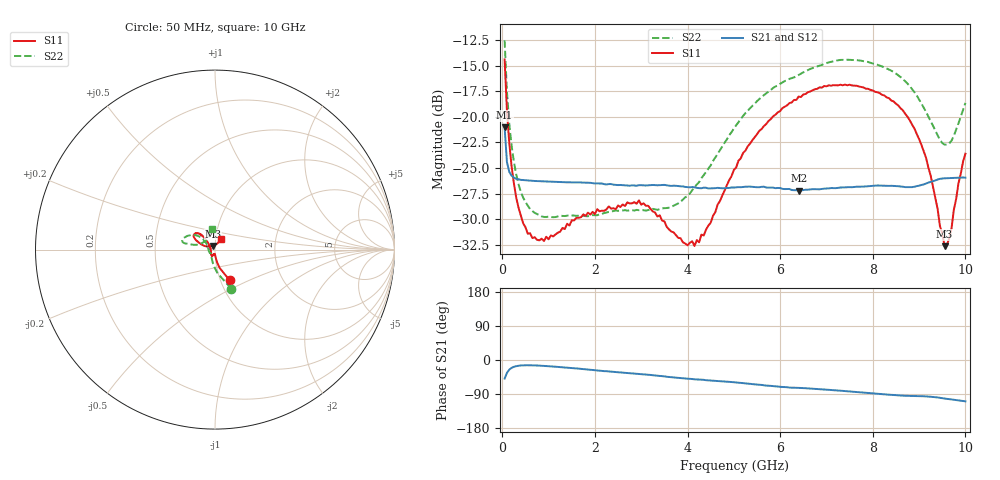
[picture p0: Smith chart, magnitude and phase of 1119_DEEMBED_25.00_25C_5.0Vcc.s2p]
!Hittite Microwave Corp.
!Digital Attenuator/PhaseShifter Rev 1.4.0
!Filename: C:\DATA\DATA\1119_DEEMBED_25.00_25C_5.0Vcc.s2p
!VNA ID: Agilent Technologies,N5224A,MY51441122,A.10.45.03
!Device type:
!2 Port Calibration.
!Temp(C): 25
!Lot Number:
!Serial Number:
!Operator:
!Misc:
!Attenuator:  25.000
# GHZ S DB R 50.0
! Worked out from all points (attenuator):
!   200 points, 50 MHz to 10 GHz, reference 50 ohm
!   highest |S21| = -21.02 dB at 50 MHz (marker M1); lowest = -27.2 dB at 6.4 GHz (marker M2)
!   lowest |S11| = -32.6 dB at 9.55 GHz (marker M3), VSWR 1.05, Z = 48.8 + j1.96 ohm
!   |S11| at or under -10 dB: start of sweep to end of sweep
!   |S22| runs from -29.8 to -12.6 dB; largest |S21 - S12| = 0.00016
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0.05  -14.40 -64.3  -21.02 -49.0  -21.03 -49.1  -12.55 -67.3
0.1  -19.41 -75.5  -24.41 -34.1  -24.41 -34.1  -17.51 -83.9
0.2  -24.80 -82.8  -25.74 -20.8  -25.74 -20.8  -22.79 -100.5
0.35  -28.86 -86.3  -26.10 -15.2  -26.09 -15.1  -26.57 -114.6
0.55  -31.40 -90.6  -26.22 -13.8  -26.22 -13.8  -28.66 -126.3
0.9  -32.12 -96.6  -26.29 -15.6  -26.30 -15.6  -29.77 -135.7
1.75  -29.52 -111.4  -26.42 -24.0  -26.41 -24.1  -29.65 -140.6
2.95  -28.15 -117.9  -26.67 -36.6  -26.68 -36.7  -29.11 -159.8
3.4  -29.61 -130.8  -26.67 -41.9  -26.68 -42.0  -29.01 -173.4
4.15  -32.60 -177.9  -26.88 -51.0  -26.90 -51.1  -26.92 156.1
5.05  -24.94 135.2  -26.88 -59.2  -26.90 -59.2  -20.83 138.8
5.55  -21.37 132.1  -26.87 -65.2  -26.89 -65.3  -18.26 141.3
6.4  -18.02 134.6  -27.19 -73.6  -27.20 -73.7  -15.92 150.0
6.7  -17.41 137.6  -27.06 -75.8  -27.08 -75.8  -15.24 154.0
7.5  -16.87 146.1  -26.86 -83.0  -26.87 -83.1  -14.44 163.6
8.35  -18.18 152.5  -26.74 -91.5  -26.74 -91.5  -15.38 168.1
8.75  -19.99 156.4  -26.86 -94.6  -26.86 -94.6  -16.76 168.1
9.05  -22.73 160.2  -26.65 -95.4  -26.66 -95.4  -18.69 166.9
9.25  -25.73 159.5  -26.35 -96.9  -26.37 -97.0  -20.43 162.2
9.55  -32.62 120.7  -26.00 -101.7  -26.01 -101.7  -22.71 138.1
9.7  -30.91 80.1  -25.97 -104.1  -25.98 -104.0  -22.33 119.9
10  -23.60 60.6  -25.94 -109.1  -25.95 -109.1  -18.64 98.5
